(* Logix 5000 AddOnInstructionDefinition export AMCI_SV160E2_Preset_Position; software revision 20.03 *)

ADD_ON_INSTRUCTION AMCI_SV160E2_Preset_Position   (* revision 1.0, vendor AMCI, ExecuteEnableInFalse *)
// Revision note:
// 8/2019 Version 0 Initial release of SV160E2 Add On Instructions.
// 3/17/20 Version 1 replaced the generic EDS file with a more complete V1.6 EDS file.
VAR_INPUT
   Status_Word_0 : INT; {required}
        .0   // Set when the SV160E2 is moving CW
        .1   // Set when SV160E2 is moving CCW
        .7   // SV160E2 Move Complete bit
        .11   // Set when there is an input error
        .12   // set when there is a command error
        .13   // set when there is a configuration error
   Status_Word_1 : INT; {required}
        .15   // Set when SV160E2 is enabled
   save_in_flash_0_no_1_yes : BOOL; {required}
   Target_Position : DINT; {required}
END_VAR
VAR_IN_OUT
   AMCI_SV160E2_output_data : _000A:SV160E2_9125ACD4:O:0; {required}
END_VAR
VAR_OUTPUT
   EN : BOOL; {visible}
END_VAR
VAR
   command_data_block : INT[10];
        [0]   // Command Word 0
        [1]   // Command Word 1
        [2]   // Upper Target Position
        [3]   // Lower Target Position
        [5]   // Lower Programmed Speed
END_VAR

ROUTINE EnableInFalse   (* ladder *)
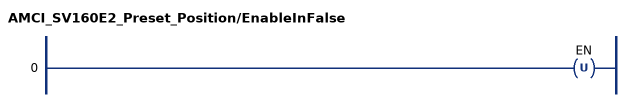
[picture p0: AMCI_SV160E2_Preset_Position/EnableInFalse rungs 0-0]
   0: OTU(EN);
END_ROUTINE

ROUTINE Logic   (* ladder *)
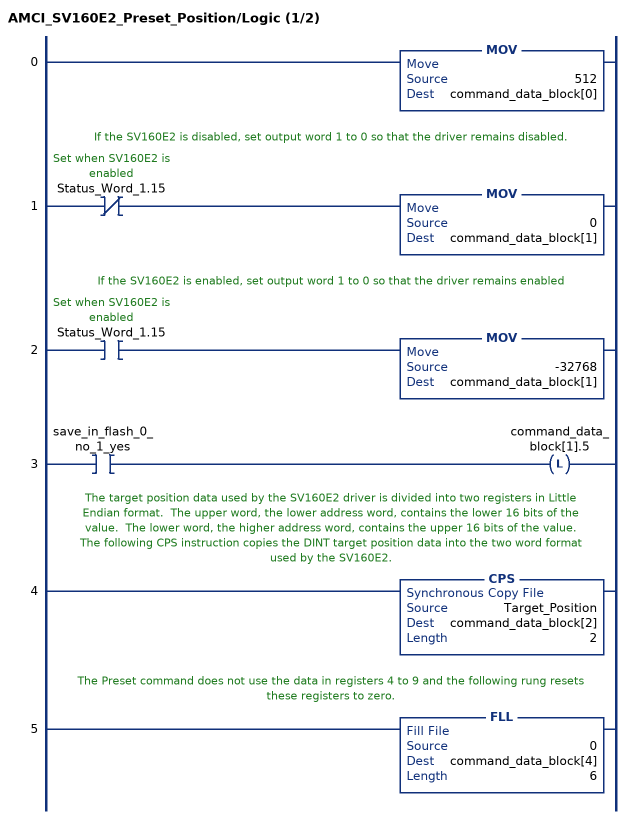
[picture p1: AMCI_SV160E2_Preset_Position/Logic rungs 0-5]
   0: MOV(512,command_data_block[0]);
   // If the SV160E2 is disabled, set output word 1 to 0 so that the driver remains disabled.
   1: XIO(Status_Word_1.15)MOV(0,command_data_block[1]);
   // If the SV160E2 is enabled, set output word 1 to 0 so that the driver remains enabled
   2: XIC(Status_Word_1.15)MOV(-32768,command_data_block[1]);
   3: XIC(save_in_flash_0_no_1_yes)OTL(command_data_block[1].5);
   // The target position data used by the SV160E2 driver is divided into two registers in Little Endian format.  The upper word, the lower address word, contains the lower 16 bits of the value.  The lower word, the higher address word, contains the upper 16 bits of the value.
   // The following CPS instruction copies the DINT target position data into the two word format used by the SV160E2.
   4: CPS(Target_Position,command_data_block[2],2);
   // The Preset command does not use the data in registers 4 to 9 and the following rung resets these registers to zero.
   5: FLL(0,command_data_block[4],6);
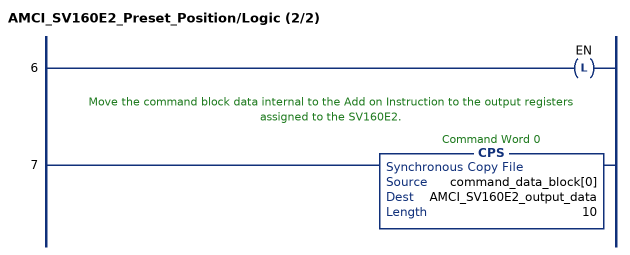
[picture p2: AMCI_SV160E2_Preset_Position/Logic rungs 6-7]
   6: OTL(EN);
   // Move the command block data internal to the Add on Instruction to the output registers assigned to the SV160E2.
   7: CPS(command_data_block[0],AMCI_SV160E2_output_data,10);
END_ROUTINE
END_ADD_ON_INSTRUCTION
